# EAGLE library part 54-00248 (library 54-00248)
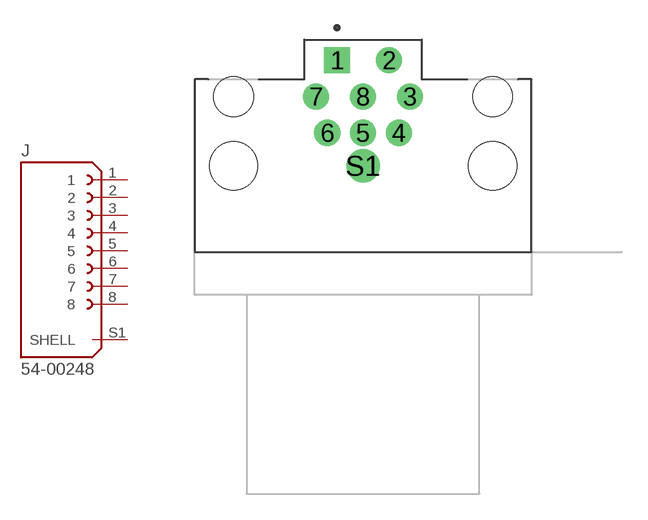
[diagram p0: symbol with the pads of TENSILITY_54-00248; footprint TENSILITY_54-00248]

Designator prefix J

## 54-00248 (MANUFACTURER: Tensility; MAXIMUM_PACKAGE_HEIGHT: 16mm; PARTREV: A1; STANDARD: Manufacturer Recommendations)  [TENSILITY_54-00248]
1  1  pas
2  2  pas
3  3  pas
4  4  pas
5  5  pas
6  6  pas
7  7  pas
8  8  pas
S1  SHELL  pas

## Footprint TENSILITY_54-00248 (pad centres in mm)
drill 1 pad 1.4 square: 1 -1.5,2.1
drill 1 pad 1.4: 2 1.5,2.1; 3 2.725,0; 4 2.075,-2.1; 5 0,-2.1; 6 -2.075,-2.1; 7 -2.725,0; 8 0,0
drill 1.3 pad 1.7: S1 0,-4
hole 2.3 at -7.5,0
hole 2.8 at -7.5,-4
hole 2.3 at 7.5,0
hole 2.8 at 7.5,-4

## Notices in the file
This work is licensed under a Creative Commons Attribution-ShareAlike 4.0 International License (CC BY-SA) with Design Exception 1.0
